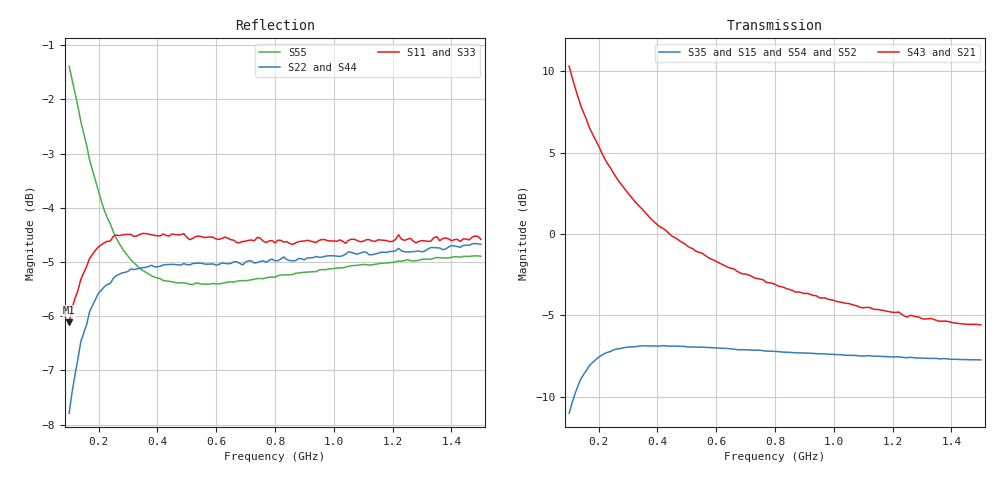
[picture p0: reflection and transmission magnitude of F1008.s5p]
!  POLYFET RF DEVICES
!  S PARAMETERS FOR
!  F1008 (Each Side)
!  VDS=28, IDQ=400mA
! Date: Mon Oct 21 17:59:02 1991
! Bias (V mA) : V1=2.0480000  I1=0.0039989  V2=27.998000  I2=408.05560
!AWR Design Environment (2053) Wed Feb 04 14:26:26 2004
!freq-unit  param-type  data-format  keyword  impedance-ohms
# MHz  S  MA  R  50
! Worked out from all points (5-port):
!   141 points, 100 MHz to 1.5 GHz, reference 50 ohm
!   strongest paths, dB at 100 MHz, 450 MHz, 800 MHz, 1.15 GHz, 1.5 GHz:
!     S43: 10.3, -0.1, -3.1, -4.6, -5.6
!     S21: 10.3, -0.1, -3.1, -4.6, -5.6
!     S35: -11.0, -6.9, -7.2, -7.5, -7.7
!     S15: -11.0, -6.9, -7.2, -7.5, -7.7
!     S54: -11.0, -7.2, -7.4, -7.5, -7.6
!     S52: -11.0, -7.2, -7.4, -7.5, -7.6
!   lowest |S11| = -6.1 dB at 100 MHz (marker M1), VSWR 2.96, Z = 27.6 - j35.9 ohm
!   |S11| at or under -10 dB: nowhere
